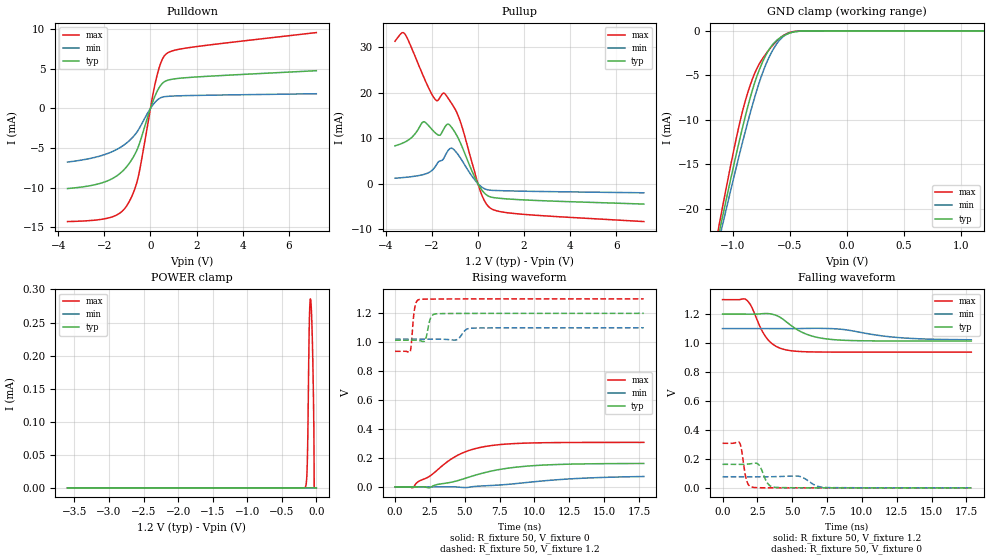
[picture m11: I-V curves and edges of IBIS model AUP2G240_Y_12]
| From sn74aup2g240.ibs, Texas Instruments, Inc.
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[Model]   AUP2G240_Y_12
Model_type  3-state
Enable   Active-Low
Vref =   0
Rref =   1E6
Cref =   30p
Vmeas =   0.6
| variable   typ   min   max
C_comp   2.19pF   1.99pF   2.49pF
| C_pullup   2.86pF   2.20pF   3.52pF
| C_pulldown   2.55pF   2.26pF   2.92pF
| C_tri-state   2.19pF   1.99pF   2.49pF
[Temperature Range]   40   100   -40
| Ambient temperature   25   85   -40
[Voltage range]   1.2   1.1   1.3
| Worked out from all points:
|   slope of the pulldown table from 0 to 0.18 V, typ, clamps not added: 125 ohm
|   slope of the pullup table from 0 to 0.18 V, typ, clamps not added: 124 ohm
|   GND clamp passes 1 mA (typ) near -0.61 V on its own axis
|   rising waveform, R_fixture 50, V_fixture 0: 20-80 % time 4.08ns typ, 5.26ns min, 2.88ns max; typ from 0 V to 0.162 V
|   falling waveform, R_fixture 50, V_fixture 1.2: 20-80 % time 1.96ns typ, 3.29ns min, 1.2ns max; typ from 1.2 V to 1.01 V
|   rising waveform, R_fixture 50, V_fixture 1.2: 20-80 % time 256ps typ, 378ps min, 209ps max; typ from 1.01 V to 1.2 V
|   falling waveform, R_fixture 50, V_fixture 0: 20-80 % time 447ps typ, 756ps min, 305ps max; typ from 0.163 V to 0 V
[GND Clamp]
| AUP2G240_Y_12
|   Voltage   I(typ)   I(min)   I(max)
-3.6V     -191.7mA   -177.9mA   -208.5mA
-1.13V    -23.31mA   -24.02mA   -22.49mA
-1.105V   -21.79mA   -22.63mA   -20.79mA
-1.085V   -20.58mA   -21.53mA   -19.44mA
-955mV    -13.03mA   -14.56mA   -11.2mA
-855mV    -7.853mA   -9.579mA   -6.382mA
-790mV    -5.135mA   -6.676mA   -4.254mA
-720mV    -2.969mA   -4.074mA   -2.762mA
-590mV    -820.1uA   -1.043mA   -839.7uA
-510mV    -284.1uA   -282.5uA   -216.8uA
-400mV    -28.32uA   -30.86uA   -11.42uA
1.2V      123.1pA    18.2nA     21.35pA
[POWER Clamp]
| AUP2G240_Y_12
|   Voltage   I(typ)   I(min)   I(max)
-3.6V     1.486nA    2.958nA    506.1pA
-165mV    871pA      3.28nA     458.8nA
-145mV    2.374nA    5.515nA    6.95uA
-130mV    7.466nA    8.889nA    38.54uA
-120mV    17.34nA    12.03nA    99.49uA
-100mV    78.07nA    18.2nA     255uA
-85mV     147.2nA    18.27nA    285.8uA
-70mV     137.2nA    13.55nA    266.3uA
-50mV     31.64nA    5.638nA    189.1uA
-35mV     1.152nA    2.45nA     83.83uA
-30mV     350.8pA    1.86nA     29.77pA
0V        0A         0A         0A
[Pulldown]
| AUP2G240_Y_12
|   Voltage   I(typ)   I(min)   I(max)
-3.6V     -10.11mA   -6.771mA   -14.28mA
-1.735V   -8.977mA   -5.551mA   -13.76mA
-1.285V   -8.113mA   -4.879mA   -13.12mA
-970mV    -7.13mA    -4.204mA   -12.01mA
-710mV    -5.964mA   -3.444mA   -10.41mA
-525mV    -4.814mA   -2.711mA   -8.581mA
90mV      761.5uA    381.6uA    1.487mA
295mV     2.185mA    1.055mA    4.264mA
495mV     3.092mA    1.407mA    6.07mA
700mV     3.505mA    1.511mA    6.919mA
1.785V    3.931mA    1.63mA     7.723mA
7.2V      4.761mA    1.852mA    9.574mA
[Pullup]
| AUP2G240_Y_12
|   Voltage   I(typ)   I(min)   I(max)
-3.6V     8.305mA    1.205mA    31.28mA
-3.19V    9.095mA    1.374mA    32.97mA
-2.375V   13.58mA    2mA        23.66mA
-1.92V    11.5mA     3.31mA     18.95mA
-1.65V    10.65mA    4.981mA    18.93mA
-1.475V   12.1mA     5.666mA    19.89mA
-1.265V   13.04mA    7.483mA    18.54mA
-1.085V   11.95mA    7.654mA    17.16mA
-770mV    9.06mA     5.712mA    13.72mA
140mV     -1.176mA   -642.2uA   -2.126mA
530mV     -2.881mA   -1.424mA   -5.332mA
7.2V      -4.469mA   -1.996mA   -8.31mA
[Ramp]
| AUP2G240_Y_12
| variable   typ   min   max
dV/dt_r   0.10/4.28E-09   0.05/5.70E-09   0.19/2.95E-09
dV/dt_f   0.11/1.98E-09   0.05/3.32E-09   0.22/1.21E-09
R_load = 50
[Rising Waveform]
| AUP2G240_Y_12
R_fixture =   50
C_fixture =   0
L_fixture =   0
V_fixture =   0
V_fixture_min = 0
V_fixture_max = 0
|   Time   V(typ)   V(min)   V(max)
0s        5.831nV    23.95nV    441.9pV
1.301ns   -8.642uV   -3.673uV   -4.417mV
1.649ns   221.1uV    -7.389uV   35.38mV
2.445ns   -6.299mV   -8.025uV   71.57mV
4.353ns   39.63mV    -80.17uV   211.5mV
5.245ns   65.87mV    -3.091mV   249.9mV
6.433ns   98.88mV    7.543mV    278.8mV
8.325ns   132.3mV    19.6mV     298.3mV
10.44ns   149.9mV    39.99mV    305.1mV
17.85ns   162mV      71.87mV    307.8mV
[Falling Waveform]
| AUP2G240_Y_12
R_fixture =   50
C_fixture =   0
L_fixture =   0
V_fixture =   1.2
V_fixture_min = 1.1
V_fixture_max = 1.3
|   Time   V(typ)   V(min)   V(max)
0s        1.2V       1.1V       1.3V
1.689ns   1.2V       1.1V       1.3V
2.045ns   1.2V       1.1V       1.258V
3.157ns   1.204V     1.1V       1.036V
3.749ns   1.195V     1.1V       982.7mV
4.521ns   1.151V     1.1V       953.7mV
6.021ns   1.061V     1.101V     939.8mV
7.733ns   1.026V     1.1V       937.8mV
12.64ns   1.014V     1.038V     937.5mV
17.85ns   1.014V     1.023V     937.4mV
[Rising Waveform]
| AUP2G240_Y_12
R_fixture =   50
C_fixture =   0
L_fixture =   0
V_fixture =   1.2
V_fixture_min = 1.1
V_fixture_max = 1.3
|   Time   V(typ)   V(min)   V(max)
0s        1.014V     1.022V     937.3mV
1.101ns   1.014V     1.022V     938.4mV
1.413ns   1.014V     1.022V     1.236V
1.765ns   1.011V     1.022V     1.296V
2.145ns   1.012V     1.022V     1.298V
2.549ns   1.167V     1.022V     1.298V
2.949ns   1.197V     1.022V     1.299V
4.405ns   1.199V     1.017V     1.3V
5.561ns   1.199V     1.098V     1.3V
17.85ns   1.2V       1.1V       1.3V
[Falling Waveform]
| AUP2G240_Y_12
R_fixture =   50
C_fixture =   0
L_fixture =   0
V_fixture =   0
V_fixture_min = 0
V_fixture_max = 0
|   Time   V(typ)   V(min)   V(max)
0s        162.6mV    76.67mV    307.8mV
1.217ns   162.3mV    76.65mV    312.8mV
1.733ns   163.4mV    76.58mV    49.74mV
2.169ns   168.5mV    76.53mV    3.776mV
2.601ns   159.9mV    76.46mV    1.038mV
3.229ns   32.17mV    76.44mV    281.1uV
3.749ns   3.885mV    77.26mV    120.2uV
5.509ns   368.9uV    79.44mV    10.45uV
7.357ns   63.13uV    2.604mV    939.5nV
17.85ns   57.36nV    10.32uV    17.56nV
